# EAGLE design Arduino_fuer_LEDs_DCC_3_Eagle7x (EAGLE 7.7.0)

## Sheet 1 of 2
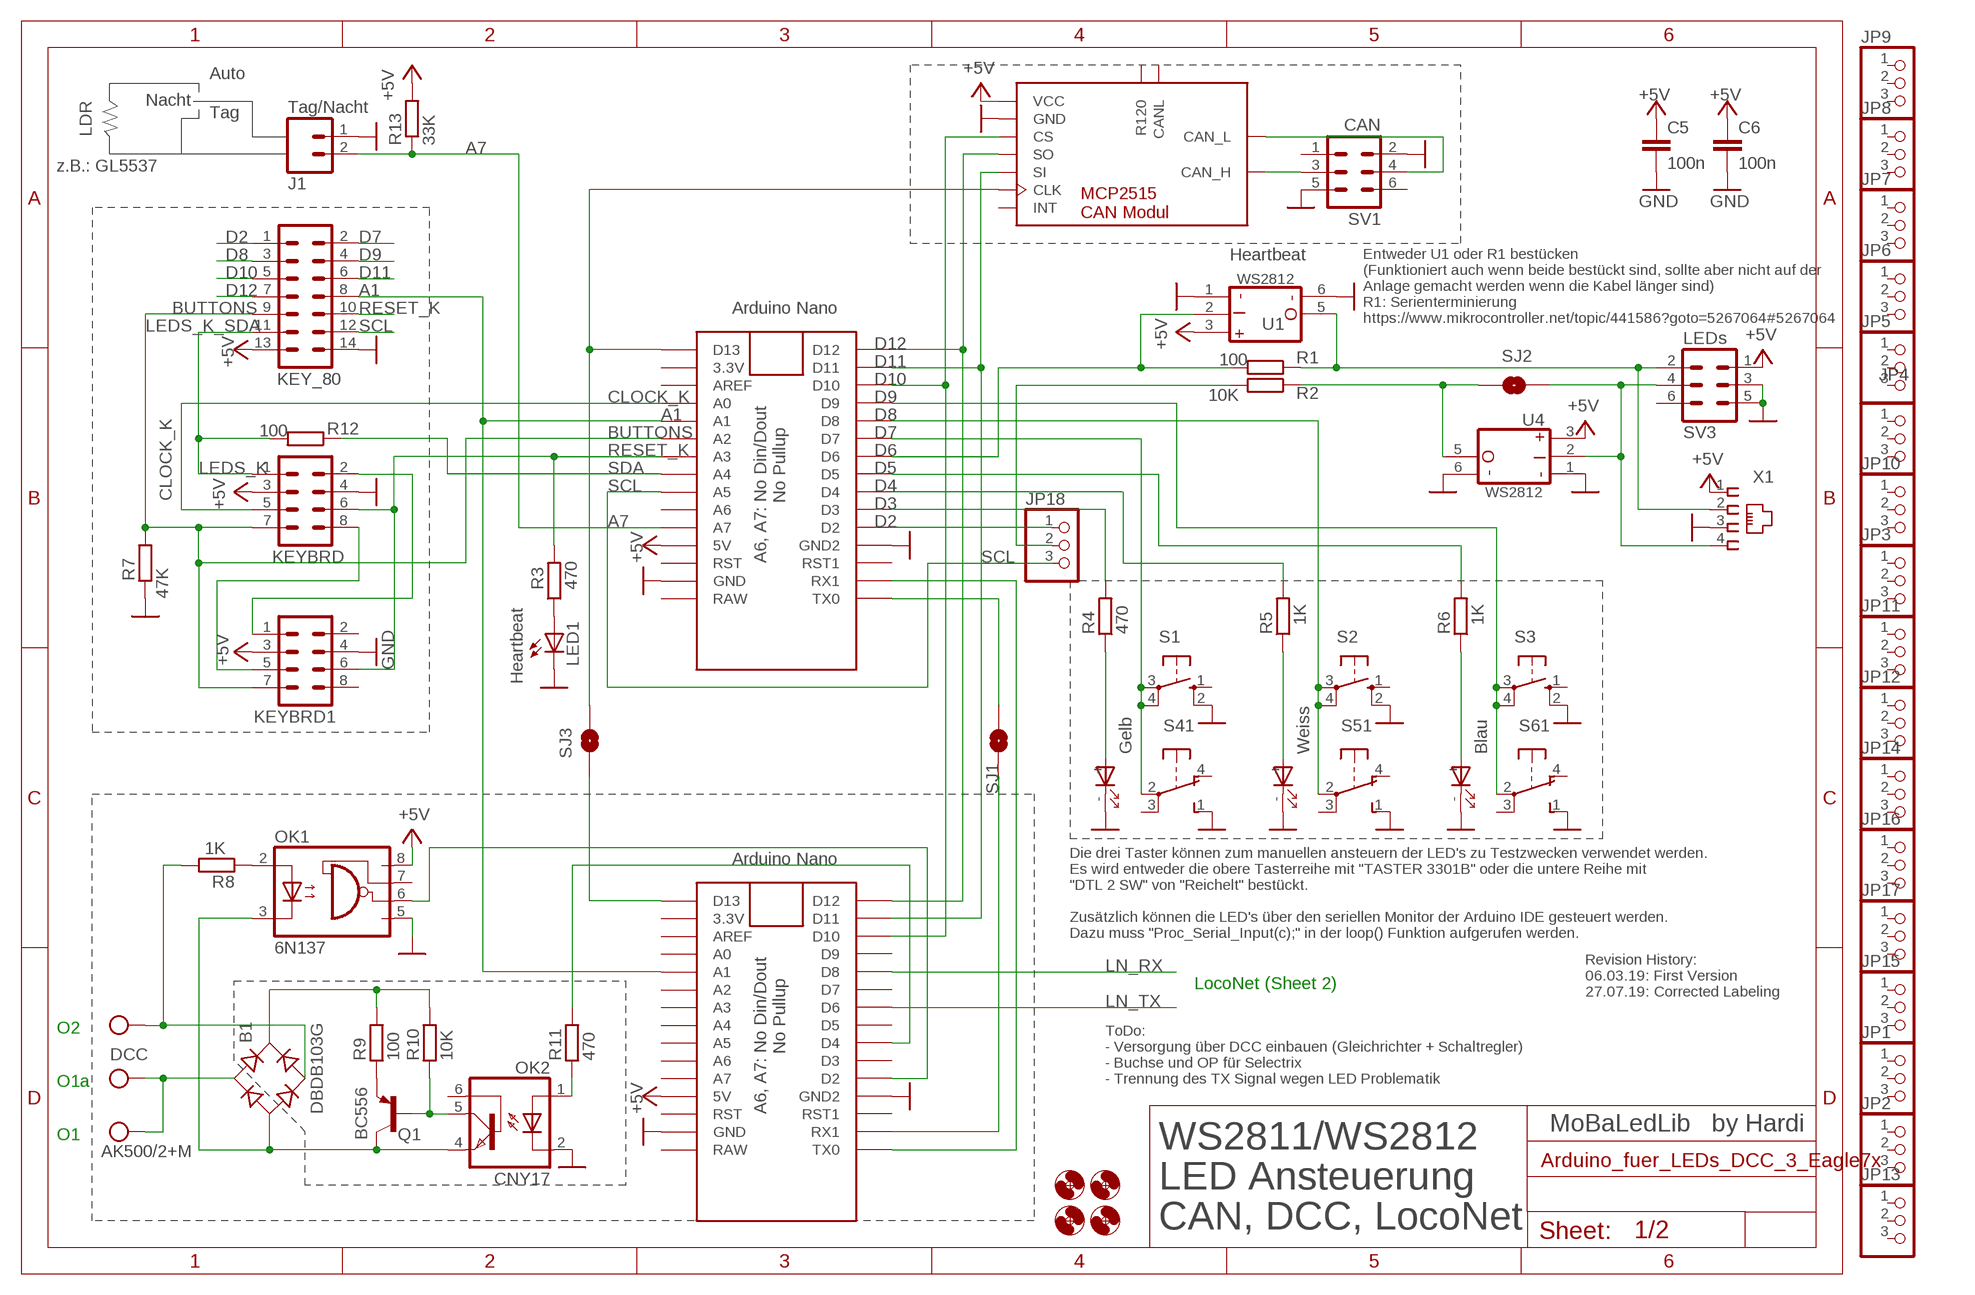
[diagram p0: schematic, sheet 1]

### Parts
B1  DBDB103G  DBDB10G  [DB]
C5  100n  C-EU025-025X050  [C025-025X050]
C6  100n  C-EU025-025X050  [C025-025X050]
CAN2  MCP2515_CAN_MODUL  [MCP2515_CAN_MODUL]
H1  MOUNT-HOLE3.0  [3,0]
H2  MOUNT-HOLE3.0  [3,0]
H3  MOUNT-HOLE3.0  [3,0]
H4  MOUNT-HOLE3.0  [3,0]
J1  Tag/Nacht  M02PTH  [1X02]
JP1  PINHD-1X3CB  [1X03-CLEANBIG]
JP2  PINHD-1X3CB  [1X03-CLEANBIG]
JP3  PINHD-1X3CB  [1X03-CLEANBIG]
JP4  PINHD-1X3CB  [1X03-CLEANBIG]
JP5  PINHD-1X3CB  [1X03-CLEANBIG]
JP6  PINHD-1X3CB  [1X03-CLEANBIG]
JP7  PINHD-1X3CB  [1X03-CLEANBIG]
JP8  PINHD-1X3CB  [1X03-CLEANBIG]
JP9  PINHD-1X3CB  [1X03-CLEANBIG]
JP10  PINHD-1X3CB  [1X03-CLEANBIG]
JP11  PINHD-1X3CB  [1X03-CLEANBIG]
JP12  PINHD-1X3CB  [1X03-CLEANBIG]
JP13  PINHD-1X3CB  [1X03-CLEANBIG]
JP14  PINHD-1X3CB  [1X03-CLEANBIG]
JP15  PINHD-1X3CB  [1X03-CLEANBIG]
JP16  PINHD-1X3CB  [1X03-CLEANBIG]
JP17  PINHD-1X3CB  [1X03-CLEANBIG]
JP18  PINHD-1X3CB  [1X03-CLEANBIG]
KEY_80  ML14  [ML14]
KEYBRD  CON-HARTING-ML_ML08  [CON-HARTING-ML_ML08]
KEYBRD1  CON-HARTING-ML_ML08  [CON-HARTING-ML_ML08]
LED1  Heartbeat  LED3MM  [LED3MM]
OK1  6N137  [DIL08]
OK2  CNY17  [DIL06]
Q1  BC556  [TO92-EBC]
R1  100  R0204/7  [0204/7]
R2  10K  R0204/7  [0204/7]
R3  470  R0204/7  [0204/7]
R4  470  R0204/7  [0204/7]
R5  1K  R0204/7  [0204/7]
R6  1K  R0204/7  [0204/7]
R7  47K  R0204/7  [0204/7]
R8  1K  R0204/7  [0204/7]
R9  100  R0204/7  [0204/7]
R10  10K  R0204/7  [0204/7]
R11  470  R0204/7  [0204/7]
R12  100  R0204/7  [0204/7]
R13  33K  R0204/7  [0204/7]
S1  10-XX  [B3F-10XX]
S2  10-XX  [B3F-10XX]
S3  10-XX  [B3F-10XX]
S4  Gelb  SRKL  [SRKL]
S5  Weiss  SRKL  [SRKL]
S6  Blau  SRKL  [SRKL]
SJ1  SOLDERJUMPERNO  [SJ_2S-NO]
SJ2  SOLDERJUMPERNO  [SJ_2S-NO]
SJ3  SOLDERJUMPERNO  [SJ_2S-NO]
SV1  CAN  ML6  [ML6]
SV3  LEDs  ML6  [ML6]
U1  WS2812_MODUL  [WS2812_LED_MODUL]
U2  LED NANO  NANO  [NANO]
U3  DCC NANO  NANO  [NANO]
U4  WS2812_MODUL  [WS2812_LED_MODUL]
X1  RJ10  [RJ10]
X2  AK500/2+M  [AK500/2+M]

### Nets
+5V: C5.1 C6.1 CAN2.1(VCC) KEY_80.13 KEYBRD1.3 KEYBRD.3 OK1.8(VCC) R13.2 SV3.1 U1.3(VDD) U2.5V U3.5V U4.3(VDD) X1.1 ; also sheet 2
A1: KEY_80.8 U2.A1 U3.A1
A7: J1.2 R13.1 U2.A7
BUTTONS: KEY_80.9 KEYBRD1.7 KEYBRD.7 R7.2 U2.A2
CAN_H: CAN2.9(CAN_H) SV1.3
CAN_L: CAN2.8(CAN_L) SV1.4
CLOCK_K: KEYBRD.5 U2.A0
D2: JP18.1 KEY_80.1 U2.D2
D3: R4.2 U2.D3
D4: R5.2 U2.D4
D5: R6.2 U2.D5
D6: R1.2 U1.2(DIN) U2.D6
D7: KEY_80.2 S1.3(P) S1.4(P1) S4.2(1:P) U2.D7
D8: KEY_80.3 S2.3(P) S2.4(P1) S5.2(1:P) U2.D8
D9: KEY_80.4 S3.3(P) S3.4(P1) S6.2(1:P) U2.D9
D10: CAN2.3(CS) KEY_80.5 U2.D10 U3.D10
D11: CAN2.5(SI) KEY_80.6 U2.D11 U3.D11
D12: CAN2.4(SO) KEY_80.7 U2.D12 U3.D12
GND: C5.2 C6.2 CAN2.2(GND) J1.1 KEY_80.14 KEYBRD1.4 KEYBRD.4 LED1.K(C) OK1.5(GND) OK2.2(C) R7.1 S1.2(S1) S2.2(S1) S3.2(S1) S4.1(1:S) S4.-(D1:C) S5.1(1:S) S5.-(D1:C) S6.1(1:S) S6.-(D1:C) SV1.2 SV1.5 SV3.3 SV3.5 U1.1(GND) U1.6(GND1) U2.GND U2.GND1(GND2) U3.GND U3.GND1(GND2) U4.1(GND) U4.6(GND1) X1.3 ; also sheet 2
LEDS_K_SDA: KEY_80.11 KEYBRD.1 R12.2
LN_RX: U3.D8 ; also sheet 2
LN_TX: U3.D6 ; also sheet 2
N$1: SJ1.2 U2.TX0
N$2: R1.1 SV3.2 U1.5(DO) X1.2
N$3: U2.RX1 U3.TX0
N$4: R4.1 S4.+(D1:A)
N$5: CAN2.6(CLK) SJ3.2 U2.D13
N$6: R5.1 S5.+(D1:A)
N$7: R6.1 S6.+(D1:A)
N$8: OK1.6(VO) U3.D2
N$9: Q1.E R9.1
N$10: OK2.5(COL) Q1.B R10.1
N$11: SJ2.1 SV3.4 U4.2(DIN) X1.4
N$12: B1.AC2 R8.2 X2.2
N$13: B1.AC1 X2.1 X2.M
N$14: B1.+ R9.2 R10.2
N$15: OK2.1(A) R11.1
N$16: R11.2 U3.D4
N$17: B1.- OK1.3(C) OK2.4(EMI) Q1.C
N$18: SJ1.1 U3.RX1
N$19: LED1.A R3.1
N$20: SJ3.1 U3.D13
N$21: OK1.2(A) R8.1
N$22: R2.1 SJ2.2 U4.5(DO)
N$24: KEYBRD1.1 KEYBRD.2
N$25: KEYBRD1.5 KEYBRD.8
N$26: JP18.2 R2.2
RESET_K: KEY_80.10 KEYBRD1.6 KEYBRD.6 R3.2 U2.A3
SCL: JP18.3 KEY_80.12 U2.A5
SDA: R12.1 U2.A4
Unconnected: CAN2.7(INT) CAN2.10(R120) CAN2.11(CANL) JP1.1 JP1.2 JP1.3 JP2.1 JP2.2 JP2.3 JP3.1 JP3.2 JP3.3 JP4.1 JP4.2 JP4.3 JP5.1 JP5.2 JP5.3 JP6.1 JP6.2 JP6.3 JP7.1 JP7.2 JP7.3 JP8.1 JP8.2 JP8.3 JP9.1 JP9.2 JP9.3 JP10.1 JP10.2 JP10.3 JP11.1 JP11.2 JP11.3 JP12.1 JP12.2 JP12.3 JP13.1 JP13.2 JP13.3 JP14.1 JP14.2 JP14.3 JP15.1 JP15.2 JP15.3 JP16.1 JP16.2 JP16.3 JP17.1 JP17.2 JP17.3 KEYBRD1.2 KEYBRD1.8 OK1.7(VE) OK2.6(BAS) S1.1(S) S2.1(S) S3.1(S) S4.3(1:P) S4.4(1:O) S5.3(1:P) S5.4(1:O) S6.3(1:P) S6.4(1:O) SV1.1 SV1.6 SV3.6 U2.3.3V U2.A6 U2.AREF U2.RAW U2.RST U2.RST1 U3.3.3V U3.A0 U3.A2 U3.A3 U3.A4 U3.A5 U3.A6 U3.A7 U3.AREF U3.D3 U3.D5 U3.D7 U3.D9 U3.RAW U3.RST U3.RST1

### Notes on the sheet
- Auto
- Nacht
- Tag
- LDR
- z.B.: GL5537
- Heartbeat
- Entweder U1 oder R1 bestücken 
  (Funktioniert auch wenn beide bestückt sind, sollte aber nicht auf der 
  Anlage gemacht werden wenn die Kabel länger sind)
  R1: Serienterminierung
  https://www.mikrocontroller.net/topic/441586?goto=5267064#5267064
- LEDS_K
- A6, A7: No Din/Dout 
              No Pullup
- Die drei Taster können zum manuellen ansteuern der LED's zu Testzwecken verwendet werden. 
  Es wird entweder die obere Tasterreihe mit "TASTER 3301B" oder die untere Reihe mit 
  "DTL 2 SW" von "Reichelt" bestückt.
  
  Zusätzlich können die LED's über den seriellen Monitor der Arduino IDE gesteuert werden. 
  Dazu muss "Proc_Serial_Input(c);" in der loop() Funktion aufgerufen werden.
- Revision History:
  06.03.19: First Version
  27.07.19: Corrected Labeling
- LocoNet (Sheet 2)
- ToDo:
  - Versorgung über DCC einbauen (Gleichrichter + Schaltregler)
  - Buchse und OP für Selectrix
  - Trennung des TX Signal wegen LED Problematik
- O2
- DCC
- O1a
- A6, A7: No Din/Dout 
              No Pullup
- MoBaLedLib   by Hardi
- O1
- WS2811/WS2812
  LED Ansteuerung
  CAN, DCC, LocoNet

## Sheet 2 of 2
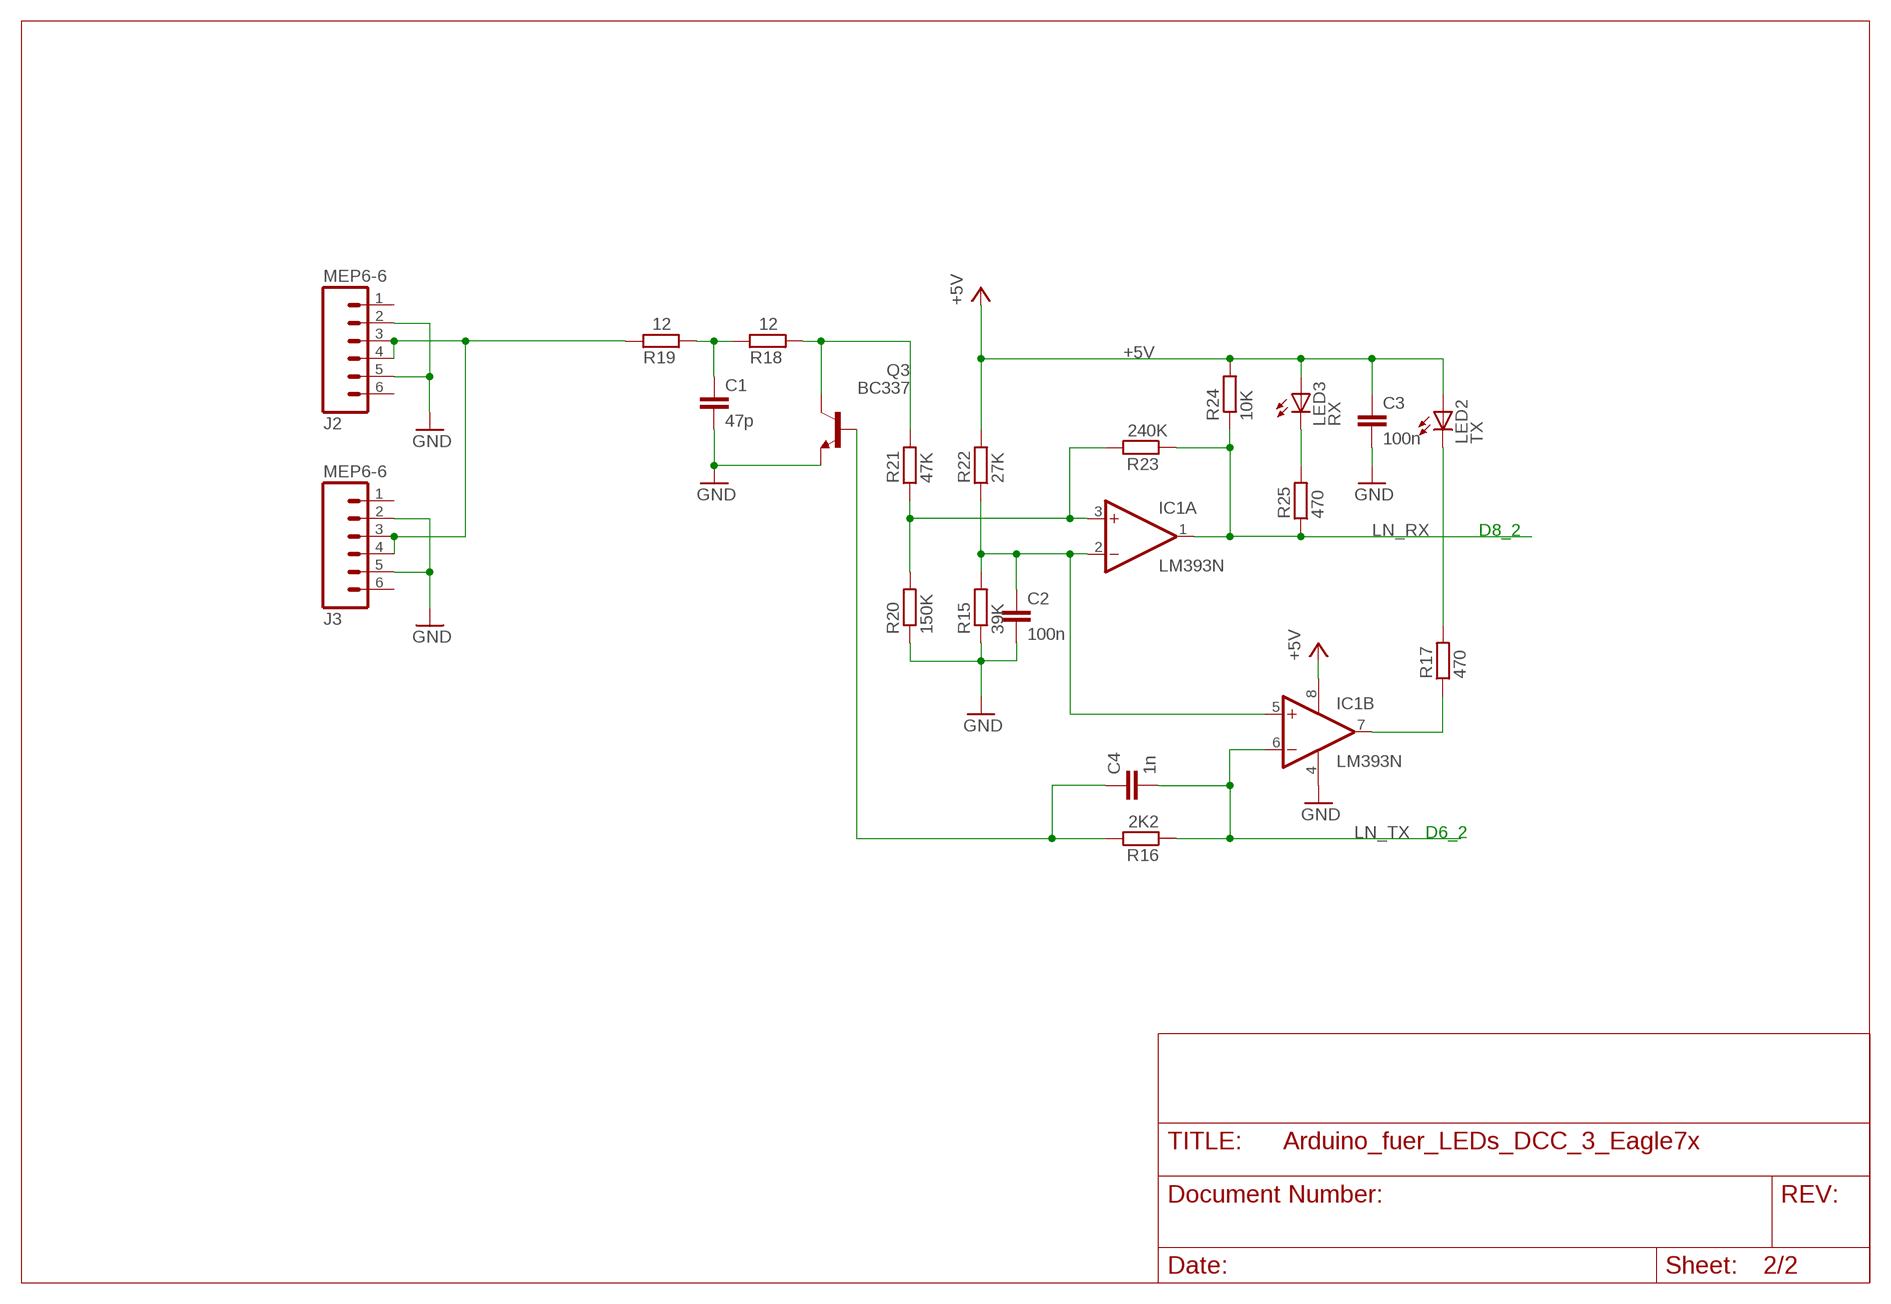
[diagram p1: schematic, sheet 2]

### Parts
C1  47p  C-EU025-025X050  [C025-025X050]
C2  100n  C-EU025-025X050  [C025-025X050]
C3  100n  C-EU025-025X050  [C025-025X050]
C4  1n  C-EU025-025X050  [C025-025X050]
IC1  LM393N  [DIL08]
J2  MEP6-6  RJ11-6PTH  [RJ11-6]
J3  MEP6-6  RJ11-6PTH  [RJ11-6]
LED2  TX  PFEIL3_LED3MM  [PFEIL3_LED3MM]
LED3  RX  PFEIL3_LED3MM  [PFEIL3_LED3MM]
Q3  BC337  [TO92]
R15  39K  R-EU_0207/2V  [0207/2V]
R16  2K2  R-EU_0207/2V  [0207/2V]
R17  470  R-EU_0207/2V  [0207/2V]
R18  12  R-EU_0207/2V  [0207/2V]
R19  12  R-EU_0207/2V  [0207/2V]
R20  150K  R-EU_0207/2V  [0207/2V]
R21  47K  R-EU_0207/2V  [0207/2V]
R22  27K  R-EU_0207/2V  [0207/2V]
R23  240K  R-EU_0207/2V  [0207/2V]
R24  10K  R-EU_0207/2V  [0207/2V]
R25  470  R-EU_0207/2V  [0207/2V]

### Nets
+5V: C3.1 IC1.8(P:V+) LED2.A LED3.A R22.2 R24.2 ; also sheet 1
GND: C1.2 C2.2 C3.2 IC1.4(P:V-) J2.2 J2.5 J3.2 J3.5 Q3.1(E) R15.1 R20.1 ; also sheet 1
LN_RX: IC1.1(A:OUT) R23.1 R24.1 R25.1 ; also sheet 1
LN_TX: C4.2 IC1.6(B:-IN) R16.1 ; also sheet 1
LOCONET: J2.3 J2.4 J3.3 J3.4 R19.1
N$31: C2.1 IC1.2(A:-IN) IC1.5(B:+IN) R15.2 R22.1
N$32: C4.1 Q3.2(B) R16.2
N$33: Q3.3(C) R18.2 R21.2
N$34: IC1.3(A:+IN) R20.2 R21.1 R23.2
N$35: IC1.7(B:OUT) R17.1
N$36: LED3.K(C) R25.2
N$37: LED2.K(C) R17.2
N$38: C1.1 R18.1 R19.2
Unconnected: J2.1 J2.6 J3.1 J3.6

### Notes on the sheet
- D8_2
- D6_2

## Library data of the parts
B1 = Arduino_fuer_LEDs_DCC_2:DB?*G: Single Phase 1.0 AMP Glass Passivated Bridge Rectifier Taiwan Semiconductor Co.,Ltd. - TSC Source: http://www.taiwansemi.com/TSCbig5/ezcatfiles/cust/img/img/db101g.pdf http://www.ts.com.tw/db/pictures/modules/PDT/PDT060207001/DBLS201G.pdf
C1-C6 = rcl:C-EU: CAPACITOR, European symbol
CAN2 = Arduino_fuer_LEDs_DCC_2_All:MCP2515_CAN_MODUL: MCP2515 CAN Modul
H1-H4 = holes:MOUNT-HOLE: MOUNTING HOLE with drill center marker
IC1 = linear:LM393: COMPARATOR
J1 = SparkFun-Connectors:M02: Standard 2-pin 0.1" header. Use with
J2 J3 = SparkFun-Connectors:RJ11-6: RJ11 Jack Simple 6 pin RJ11 jack. Commonly found on CAT3 devices and Microchip programmers. SKU: PRT-00132
JP1-JP18 = adafruit:PINHD-1X3: PIN HEADER
KEY_80 = Arduino_fuer_LEDs_DCC_2:ML14: HARTING; OC_FARNELL: unknown; OC_NEWARK: unknown
KEYBRD KEYBRD1 = PushButtonAction_4017_2:CON-HARTING-ML_ML08: Modified by Hardi; OC_FARNELL: unknown; OC_NEWARK: unknown
LED1 = Arduino_fuer_LEDs_DCC_2:LED: LED
LED2 LED3 = _relaisblock2Gl-Frontplatte:PFEIL3_LED: LED
OK1 = Arduino_fuer_LEDs_DCC_2:6N137: MOTOROLA OPTO COUPLER; MPN: 6N137; OC_FARNELL: 1328376; OC_NEWARK: 52M1895
OK2 = Arduino_fuer_LEDs_DCC_2:CNY17: SIEMENS OPTO COUPLER; MPN: CNY17-1; OC_FARNELL: 1045399; OC_NEWARK: 05M4044
Q1 = transistor-pnp:BC556*: PNP Transistror
Q3 = transistor-npn:BC337*: NPN Transistor
R1-R13 = Arduino_fuer_LEDs_DCC_2:R: RESISTOR, European symbol; SPICEMODEL: NONE; SPICEPREFIX: R
R15-R25 = rcl:R-EU_: RESISTOR, European symbol
S1-S3 = switch-omron:10-XX: OMRON SWITCH; MPN: B3F-1000; OC_FARNELL: 176432; OC_NEWARK: 36M3542
S4-S6 = switch-misc:SRKL: SWITCH
SJ1-SJ3 = SparkFun-Retired:SOLDERJUMPER: Solder Jumper
SV1 SV3 = Arduino_fuer_LEDs_DCC_2:ML6: HARTING; OC_FARNELL: unknown; OC_NEWARK: unknown
U1 U4 = Arduino_fuer_LEDs_DCC_2_All:WS2812_MODUL: WS2812 Modul mit Winkelsteckern (by Hardi)
U2 U3 = Arduino_fuer_LEDs_DCC_2:NANO: Arduino Nano
X1 = RJ10:RJ10: RJ10 Connector "C:\Dat\Märklin\Schaltpläne\Allgemein\RJ10_Stecker_Layout.docx" ...; OC_FARNELL: unknown; OC_NEWARK: unknown
X2 = Arduino_fuer_LEDs_DCC_2:AK500/2+M

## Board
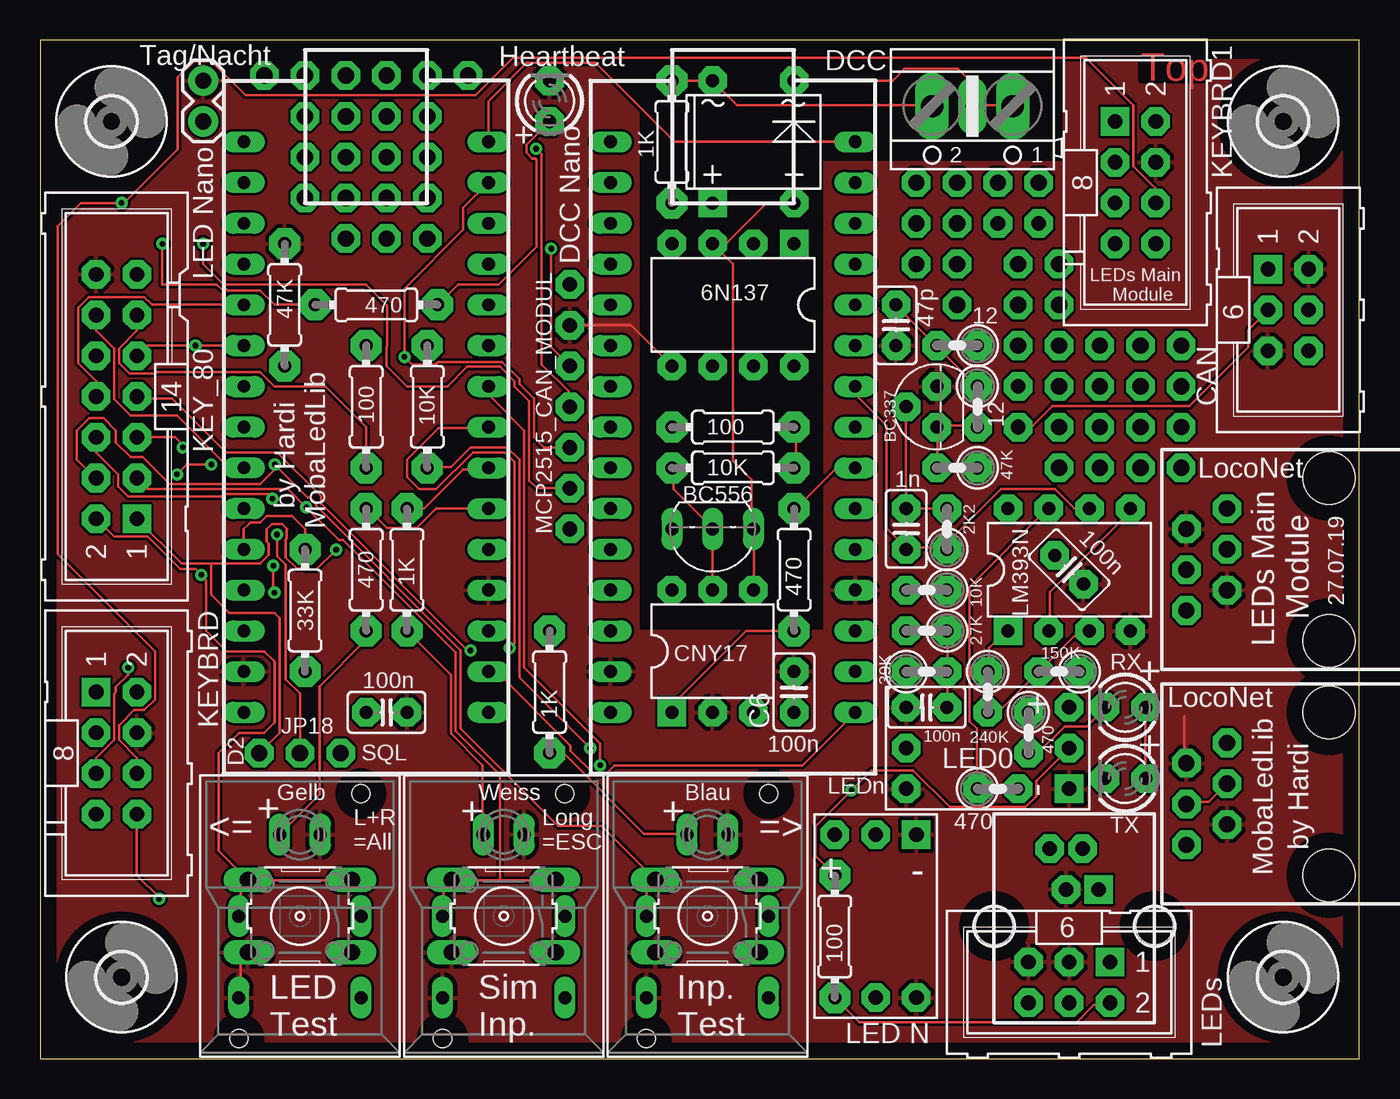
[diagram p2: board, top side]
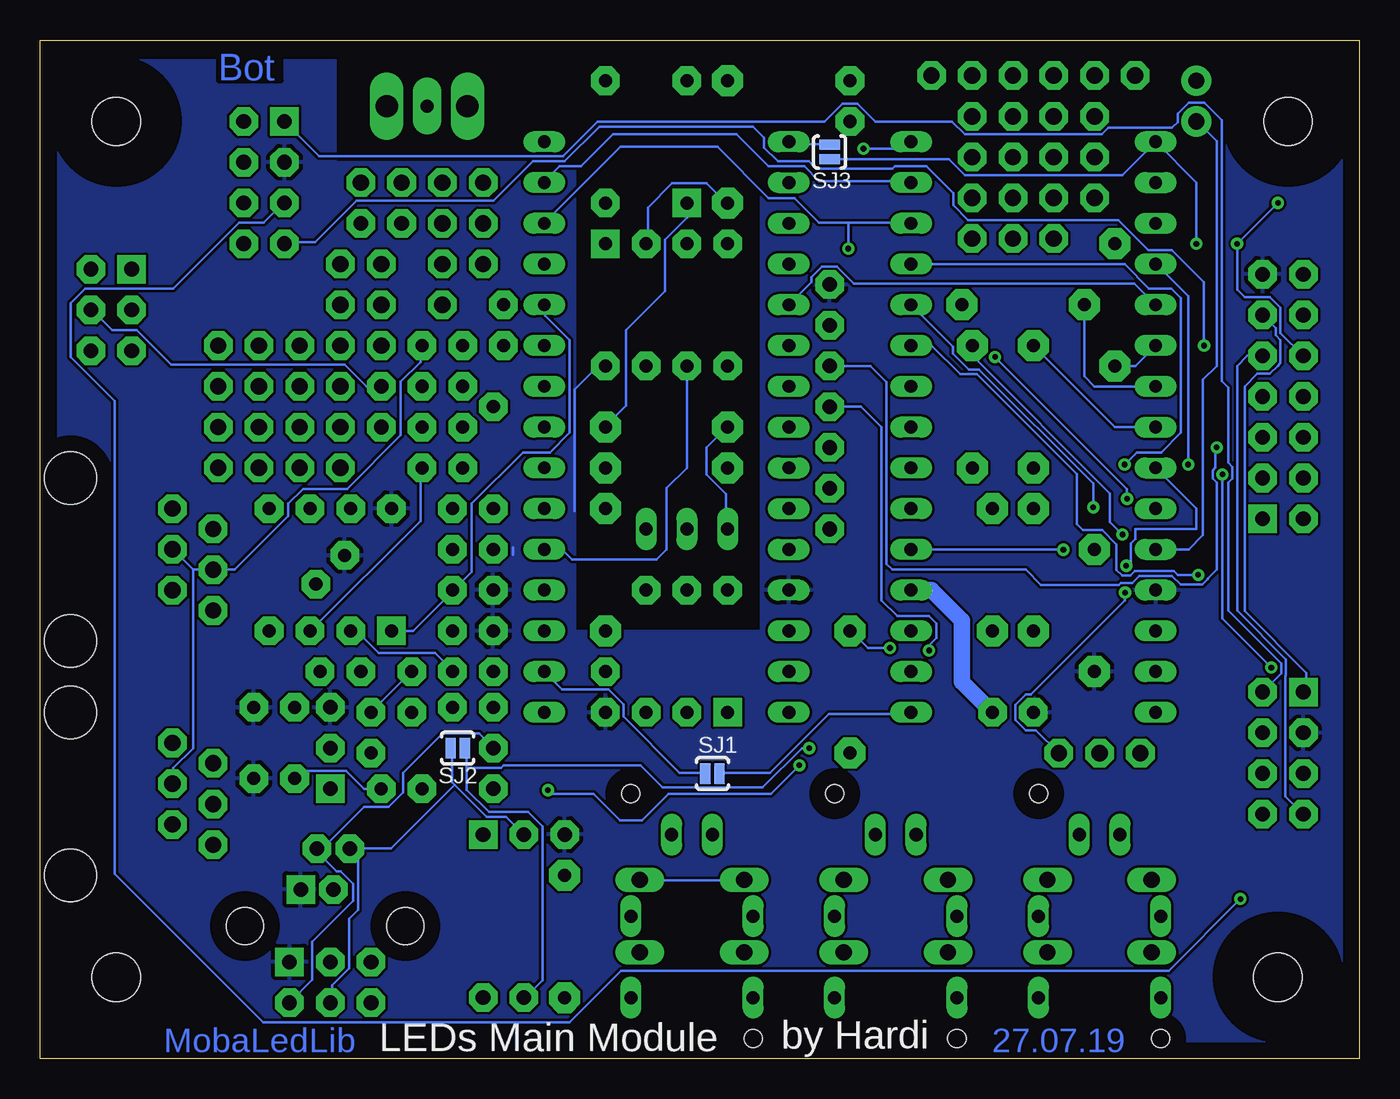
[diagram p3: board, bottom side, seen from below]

Size 82.22 x 63.49 mm. Coordinates in mm from the lower left corner, seen from the top.
Outline: 0,0 82.22,0 82.22,63.49 0,63.49 0,0
Copper layers (1*16): Top 0.035mm / dielectric 1.5mm / Bottom 0.035mm
Design rules "default": minimum track width 6mil, minimum drill 0.35mm, track to track 6mil, track to pad 6mil, pad to pad 6mil, via to via 6mil, smd to smd 6mil, copper to edge 40mil, drill to drill 6mil, minimum pad ring 10mil, minimum via ring 8mil, stop-mask expansion 4mil, vias tented up to drill 0mil, thermal gap 10mil

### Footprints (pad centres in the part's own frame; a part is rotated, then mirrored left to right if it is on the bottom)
DB = drill 0.813 pad 1.778 square: + -2.54,-3.81 | drill 0.813 pad 1.778 octagon: - 2.54,-3.81; AC1 2.54,3.81; AC2 -2.54,3.81
C025-025X050 = drill 0.813 pad 1.778 octagon: 1 -1.27,0; 2 1.27,0
MCP2515_CAN_MODUL = drill 0.914 pad 1.778 octagon: 1 0,0; 2 0,-2.54; 3 0,-5.08; 4 0,-7.62; 5 0,-10.16; 6 0,-12.7; 7 0,-15.24; 8 27.94,-6.35; 9 27.94,-8.89; 10 26.67,3.81; 11 29.21,3.81
3,0 = hole 3: 0,0
DIL08 = drill 0.813 pad 1.778 square: 1 -3.81,-3.81 | drill 0.813 pad 1.778 octagon: 2 -1.27,-3.81; 3 1.27,-3.81; 4 3.81,-3.81; 5 3.81,3.81; 6 1.27,3.81; 7 -1.27,3.81; 8 -3.81,3.81
1X02 = drill 1.016 pad 1.88: 1 0,0; 2 2.54,0
RJ11-6 = drill 1.016 pad 1.778 octagon: 1 1.905,8.89; 2 3.175,6.35; 3 4.445,8.89; 4 5.715,6.35; 5 6.985,8.89; 6 8.255,6.35 | hole 3.251: 0,0; 10.16,0
1X03-CLEANBIG = drill 1.016 pad 1.778 octagon: 1 -2.54,0; 2 0,0; 3 2.54,0
ML14 = drill 0.914 pad 1.778 square: 1 -7.62,-1.27 | drill 0.914 pad 1.778 octagon: 2 -7.62,1.27; 3 -5.08,-1.27; 4 -5.08,1.27; 5 -2.54,-1.27; 6 -2.54,1.27; 7 0,-1.27; 8 0,1.27; 9 2.54,-1.27; 10 2.54,1.27; 11 5.08,-1.27; 12 5.08,1.27; 13 7.62,-1.27; 14 7.62,1.27
CON-HARTING-ML_ML08 = drill 0.914 pad 1.778 square: 1 -5.08,-1.27 | drill 0.914 pad 1.778 octagon: 2 -5.08,1.27; 3 -2.54,-1.27; 4 -2.54,1.27; 5 0,-1.27; 6 0,1.27; 7 2.54,-1.27; 8 2.54,1.27
LED3MM = drill 0.813 pad 1.778 octagon: A -1.27,0; K 1.27,0
PFEIL3_LED3MM = drill 0.813 pad 1.778 octagon: A -1.27,0; K 1.27,0
DIL06 = drill 0.813 pad 1.778 square: 1 -2.54,-3.81 | drill 0.813 pad 1.778 octagon: 2 0,-3.81; 3 2.54,-3.81; 4 2.54,3.81; 5 0,3.81; 6 -2.54,3.81
TO92-EBC = drill 0.813 long: B 0,-1.27; C -2.54,-1.27; E 2.54,-1.27
TO92 = drill 0.813 pad 1.778 octagon: 1 1.27,0; 2 0,1.905; 3 -1.27,0
0204/7 = drill 0.813 pad 1.93 octagon: 1 -3.81,0; 2 3.81,0
0207/2V = drill 0.813 pad 1.778 octagon: 1 -1.27,0; 2 1.27,0
B3F-10XX = drill 1.016 long: 1 -3.251,2.261; 2 3.251,2.261; 3 -3.251,-2.261; 4 3.251,-2.261
SRKL = drill 0.813 long: 1 -3.81,-5.08; 2 -3.81,0; 3 3.81,0; 4 3.81,-5.08; + -1.27,5.08; - 1.27,5.08 | hole 1.118: 3.81,7.62; -3.81,-7.62
SJ_2S-NO = smd 0.635 x 1.27: 1 -0.45,0; 2 0.45,0
ML6 = drill 0.914 pad 1.778 square: 1 -2.54,-1.27 | drill 0.914 pad 1.778 octagon: 2 -2.54,1.27; 3 0,-1.27; 4 0,1.27; 5 2.54,-1.27; 6 2.54,1.27
WS2812_LED_MODUL = drill 0.914 pad 1.778 square: 1 -5.08,-5.08 | drill 0.914 pad 1.778 octagon: 2 -2.54,-5.08; 3 0,-5.08; 5 -2.54,5.08; 6 -5.08,5.08
NANO = drill 0.8 long: 3.3V -10.16,24.13; 5V -10.16,-1.27; A0 -10.16,19.05; A1 -10.16,16.51; A2 -10.16,13.97; A3 -10.16,11.43; A4 -10.16,8.89; A5 -10.16,6.35; A6 -10.16,3.81; A7 -10.16,1.27; AREF -10.16,21.59; D2 5.08,1.27; D3 5.08,3.81; D4 5.08,6.35; D5 5.08,8.89; D6 5.08,11.43; D7 5.08,13.97; D8 5.08,16.51; D9 5.08,19.05; D10 5.08,21.59; D11 5.08,24.13; D12 5.08,26.67; D13 -10.16,26.67; GND -10.16,-6.35; GND1 5.08,-1.27; RAW -10.16,-8.89; RST -10.16,-3.81; RST1 5.08,-3.81; RX1 5.08,-6.35; TX0 5.08,-8.89
RJ10 = drill 0.9 pad 1.778 square: 1 -1.524,-2.3 | drill 0.9 pad 1.778 octagon: 2 -0.508,-4.84; 3 0.508,-2.3; 4 1.524,-4.84 | hole 2.3: 5,0; -5,0
AK500/2+M = drill 1.397 long: 1 -2.515,0; 2 2.515,0 | drill 0.813 pad 1.778 long: M 0,0

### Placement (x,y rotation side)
B1  44.45,57.15 0 top
C1  53.34,45.72 270 top
C2  55.24,21.91 180 top
C3  64.14,30.48 315 top
C4  53.98,33.02 270 top
C5  21.59,21.59 0 top
C6  46.99,22.86 90 top
CAN2  33.02,48.26 0 top
H1  5.08,5.08 0 top
H2  4.45,58.42 0 top
H3  77.47,58.42 0 top
H4  77.47,5.08 0 top
IC1  64.14,30.48 0 top
J1  10.16,60.96 270 top
J2  80.33,11.43 90 top
J3  80.33,26.04 90 top
JP1  68.58,44.45 0 top
JP2  68.58,41.91 0 top
JP3  68.58,39.37 0 top
JP4  68.58,36.83 0 top
JP5  63.5,39.37 90 top
JP6  63.5,46.99 90 top
JP7  57.15,49.53 90 top
JP8  60.96,46.99 90 top
JP9  54.61,52.07 90 top
JP10  59.69,54.61 0 top
JP11  24.13,56.2 90 top
JP12  21.59,56.2 90 top
JP13  19.05,56.2 90 top
JP14  21.59,51.12 0 top
JP15  16.51,56.2 90 top
JP16  16.51,61.28 180 top
JP17  24.13,61.28 0 top
JP18  16.19,19.05 0 top
KEY_80  4.76,41.27 90 top
KEYBRD  4.76,17.78 270 top
KEYBRD1  68.26,53.34 270 top
LED1  31.75,59.69 90 top
LED2  67.63,17.46 180 top
LED3  67.63,21.91 180 top
OK1  43.18,46.99 180 top
OK2  41.91,25.4 0 top
Q1  41.91,31.75 180 top
Q3  55.88,40.64 90 top
R1  49.53,7.62 90 top
R2  24.13,40.64 90 top
R3  20.95,46.99 180 top
R4  20.32,30.48 90 top
R5  22.86,30.48 90 top
R6  31.75,22.86 90 top
R7  15.24,46.99 270 top
R8  39.37,57.15 90 top
R9  43.18,39.37 0 top
R10  43.18,36.83 0 top
R11  46.99,30.48 90 top
R12  20.32,40.64 270 top
R13  16.51,27.94 270 top
R15  55.24,24.13 0 top
R16  56.52,33.02 90 top
R17  59.69,16.83 0 top
R18  58.42,40.64 270 top
R19  57.15,44.45 180 top
R20  63.5,24.13 180 top
R21  57.15,36.83 180 top
R22  55.24,26.67 180 top
R23  59.05,22.86 270 top
R24  55.24,29.21 180 top
R25  61.59,20.32 270 top
S1  16.19,8.89 180 top
S2  28.89,8.89 180 top
S3  41.59,8.89 180 top
S4  16.19,8.89 0 top
S5  28.89,8.89 0 top
S6  41.59,8.89 0 top
SJ1  40.32,17.78 0 bottom
SJ2  56.2,19.37 0 bottom
SJ3  33.02,56.52 270 bottom
SV1  77.79,46.67 270 top
SV3  64.14,4.76 180 top
U1  59.05,21.91 90 top
U2  22.86,30.48 0 top
U3  45.72,30.48 0 top
U4  49.53,8.89 180 top
X1  64.45,8.26 180 top
X2  58.1,59.37 180 top

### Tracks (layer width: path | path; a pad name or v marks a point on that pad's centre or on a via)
+5V
  Top 0.152: LED2.A 68.89,17.53 68.89,21.79 LED3.A
  Bottom 0.152: 64.16,21.79 U1.3 | OK1.8 47.45,43.18 48.92,41.71 48.92,34.14 | 52.73,31.39 52.73,31.85
  pour Bottom: 1.27,0 81.28,0 81.28,62.23 63.82,62.23 63.82,55.88 48.9,55.88 48.9,26.67 37.31,26.67 37.31,62.23 0,62.23 0,1.27
A1
  Top 0.152: U2.A1 6.98,46.99 6.5,47.47 3.03,47.47 2.38,46.82 2.38,43.35 3.49,42.23 KEY_80.8
  Bottom 0.152: U2.A1 14.02,48.31 31.49,48.31 32.56,49.38 33.48,49.38 34.14,48.72 34.14,48.41 U3.A1
A7
  Top 0.152: U2.A7 12.7,33.02 13.02,33.34 13.09,33.41 13.72,33.41 14.13,33.81 15.72,33.81 16.51,33.02 R13.1
  Bottom 0.152: J1.2 10.06,58.37 8.89,57.2 8.89,43.18 9.75,42.32 9.75,32.63 10.64,31.75 U2.A7
BUTTONS  (via drill 0.35)
  Top 0.152: U2.A2 v9.68,44.45 6.67,44.45 KEY_80.9
  Bottom 0.152: KEYBRD1.7 66.9,50.9 65.08,50.9 62.48,53.49 53.95,53.49 51.51,55.93 49.53,55.93 47.36,58.1 37.78,58.1 37.1,57.42 37.1,56.78 36.24,55.93 34.29,55.93 33.83,55.47 29.11,55.47 28.96,55.63 26.98,55.63 25.3,53.95 25.3,53.19 24.38,52.27 15.03,52.27 13.16,50.41 11.68,50.41 9.68,48.42 v9.68,44.45 | R7.2 13.97,43.18 U2.A2 | KEYBRD.7 4.61,16.36 4.61,23.85 4.58,23.89 4.58,24.89 7.62,27.94 7.62,43.18 6.99,43.81 KEY_80.9
CAN_H
  Top 0.152: CAN2.9 60.96,39.47 61.87,39.47 63.09,40.69 71.63,40.69 75.29,44.35 75.29,45.41 76.5,46.63 SV1.3
CAN_L
  Bottom 0.152: CAN2.8 61.87,41.91 63.25,43.28 74.07,43.28 76.2,45.41 77.72,45.41 78.94,46.63 SV1.4
CLOCK_K  (via drill 0.35)
  Top 0.152: v10.67,37.03 9.14,37.03 v8.53,36.42 | v5.49,24.38 5.49,23.93 4.72,23.16 4.72,22.86 4.61,22.75 4.61,19.86 3.5,18.75 3.5,17.83 KEYBRD.5
  Bottom 0.152: v10.67,37.03 10.67,47.55 12.65,49.53 U2.A0 | v8.53,36.42 8.53,27.43 v5.49,24.38
D2  (via drill 0.35)
  Top 0.152: v18.45,31.73 17.2,30.48 16.51,30.48 16.43,30.56 16.02,30.56 15.32,31.26 15.32,32.37 15.37,32.42 15.37,32.99 15.4,33.02 15.08,33.34 14.45,33.34 14.13,33.02 14.13,32.22 14.24,32.12 14.24,31.38 13.72,30.87 10.64,30.87 | KEY_80.1 8.82,30.87 10.64,30.87 | 10.64,30.87 10.65,30.85 10.65,28.93 11.8,27.78 14.61,27.78 14.92,27.46 14.92,20.32 JP18.1
  Bottom 0.152: v18.45,31.73 18.47,31.75 U2.D2
D3
  Top 0.152: U2.D3 24.69,34.29 23.47,33.07 21.64,33.07 20.42,34.29 R4.2
D4
  Top 0.152: R5.2 23.93,34.29 26.36,36.73 27.89,36.73 U2.D4
D5  (via drill 0.35)
  Top 0.152: v29.26,25.6 29.57,25.91 29.57,37.19 28.96,37.8 26.98,37.8 24.69,35.51 23.62,35.51 22.86,36.27 22.86,37.34 24.84,39.32 27.89,39.32 U2.D5
  Bottom 0.152: v29.26,25.6 30.63,25.6 31.7,26.67 R6.2
D6  (via drill 0.35)
  Top 0.152: v34.9,18.29 34.9,19.66 30.18,24.38 30.18,39.17 28.04,41.3 28.04,41.91 U2.D6 | R1.2 48.31,12.65 48.31,14.48 v50.57,16.74 51.82,17.98 54.41,17.98 56.69,15.7 61.41,15.7 62.08,16.36 62.08,17.31 U1.2
  Bottom 0.152: v34.9,18.29 36.68,16.51 43.07,16.51 44.72,14.86 46.09,14.86 47.74,16.51 50.34,16.51 v50.57,16.74
D7  (via drill 0.35)
  Top 0.152: S4.2 12.5,8.99 12.5,10.82 12.8,11.12 S1.4 | S1.4 12.8,11.28 11.12,12.95 11.12,19.05 12.39,20.32 13.97,20.32 14.62,20.97 14.62,24.75 13.97,25.4 11.62,25.4 10.35,26.67 10.35,29.82 10,30.16 v10.04,30.16 9.68,30.52 8.73,30.52 6.72,32.54 4.61,32.54 KEY_80.2 | S1.4 12.95,11.12 19.36,11.12 S1.3
  Bottom 0.152: v10.04,30.16 11.32,30.16 11.55,30.4 14,30.4 14.28,30.12 14.78,30.12 15.14,30.47 15.14,32.07 16.02,32.94 17.23,32.94 17.62,33.34 17.62,36.44 23.84,42.66 24.88,42.66 26.67,44.45 U2.D7
D8  (via drill 0.35)
  Top 0.152: S5.2 25.15,8.99 25.15,10.67 25.6,11.12 S2.4 25.76,11.12 28.65,11.12 | 28.65,11.12 32,11.12 S2.3 | KEY_80.3 6.1,36.12 6.71,35.51 15.45,35.51 v16.59,34.37 18.63,32.33 18.89,32.33 25.91,25.31 25.91,20.42 28.65,17.68 28.65,11.12
  Bottom 0.152: v16.59,34.37 16.59,35.84 23.71,42.96 24.35,42.96 25.32,43.94 25.32,44.37 U2.D8
D9  (via drill 0.35)
  Top 0.152: 37.8,10.67 37.8,8.99 S6.2 | 37.8,10.67 38.25,11.12 S3.4 | KEY_80.4 3.35,36.27 2.29,37.34 2.29,39.17 3.05,39.93 3.96,39.93 4.72,39.17 4.72,38.41 5.64,37.49 6.4,37.49 8.08,35.81 13.72,35.81 14.63,36.73 v14.63,37.03 16.69,34.98 16.84,34.98 17.2,34.62 17.2,34.47 26.21,25.45 26.21,20.57 32.28,14.5 34.99,14.5 S3.4 | 37.8,10.67 S3.4
  Bottom 0.152: S3.3 44.81,11.12 38.41,11.12 S3.4 | U2.D9 14.63,49.53 13.11,48.01 11.73,48.01 11.12,47.4 11.12,39.01 12.34,37.8 13.87,37.8 v14.63,37.03
D10  (via drill 0.35)
  Top 0.152: v31.85,50.49 31.85,44.35 CAN2.3 | KEY_80.5 8.41,38.73 8.89,38.26 v8.89,38.1
  Bottom 0.152: 31.85,52.12 33.68,52.12 35.2,53.65 36.83,53.65 40.02,56.83 46.04,56.83 U3.D10 | 31.85,52.12 28.04,52.12 U2.D10 | v31.85,50.49 31.85,52.12 | v8.89,38.1 8.97,38.02 8.97,36.85 9.14,36.67 9.14,36.17 8.89,35.92 8.89,30.48 9.44,29.93 9.44,29.91 9.79,29.56 11.14,29.56 11.68,30.09 13.72,30.09 14.15,29.66 14.86,29.66 14.99,29.53 19.84,29.53 20.8,30.48 29.11,30.48 29.48,30.85 29.48,42.18 30.48,43.18 CAN2.3
D11  (via drill 0.35)
  Top 0.152: v14.48,34.9 14.17,35.2 11.58,35.2 11.43,35.05 5.49,35.05 4.88,35.66 4.88,36.42 3.5,37.8 3.5,38.71 KEY_80.6 | U2.D11 26.36,53.03 26.36,51.66 22.71,48.01 22.71,45.72 v22.71,43.74 23.19,43.26 24.62,43.26 24.8,43.43 26.98,43.43 28.8,43.43 29.87,42.37 29.87,42.06 30.79,41.15 30.79,38.73 31.42,38.1 CAN2.5
  Bottom 0.152: U2.D11 28.04,54.71 33.68,54.71 34.59,55.63 36.83,55.63 38.83,57.63 46.51,57.63 48.51,55.63 49.84,55.63 50.75,54.71 U3.D11 | v14.48,34.9 14.48,35.51 v22.71,43.74
D12  (via drill 0.35)
  Top 0.152: CAN2.4 32.92,40.69 32.92,41.6 31.24,43.28 31.24,56.39 v30.91,56.72 | KEY_80.7 6.1,41.15 8.23,41.15 11.58,37.8 14.78,37.8 17.5,35.08 17.5,34.59 26.64,25.45 v26.82,25.45 | U3.D12 39.53,57.15 34.6,62.08 30.33,62.08 27.94,59.69 U2.D12
  Bottom 0.152: v26.82,25.45 26.82,25.76 26.36,26.21 26.36,27.13 26.82,27.58 28.8,27.58 29.78,28.56 29.78,39.37 31.05,40.64 CAN2.4 | v30.91,56.72 28.37,56.72 U2.D12
GND
  Top 0.152: 64.77,24.23 R20.1 | 71.32,21.34 71.32,18.44 J2.5 | S4.1 12.5,3.81 12.5,6.25 12.8,6.55 S1.2 | 15.24,51.51 R7.1 | OK1.5 36.83,45.72 CAN2.2
  Bottom 1.016: U2.GND1 26.67,29.21 24.77,27.3 24.77,23.5 C5.2
  pour Top: 1.27,0 81.28,0 81.28,62.23 63.82,62.23 63.82,55.88 48.9,55.88 48.9,26.67 37.31,26.67 37.31,62.23 0,62.23 0,1.27
LEDS_K_SDA
  Top 0.152: KEY_80.11 6.03,45.4 4.92,44.28 4.92,43.35 5.57,42.7 7.14,42.7 7.23,42.79 13.72,42.79 14.6,41.91 17.78,41.91 20.32,39.37 R12.2
  Bottom 0.152: KEYBRD.1 3.31,23.05 3.31,24.06 7.15,27.9 7.15,41.91 6.36,42.7 5.57,42.7 5.09,43.18 5.08,43.18 5.08,43.19 4.92,43.35 4.92,44.81 5.22,45.11 5.22,45.54 KEY_80.11
LN_RX
  Top 0.152: R23.1 59.13,24.23 59.13,25.6 60.2,26.67 IC1.1
  Bottom 0.152: R25.1 61.57,21.64 59.13,24.08 R23.1 | U3.D8 50.75,46.94 50.75,46.33 49.23,44.81 49.23,39.01 50.44,37.8 52.12,37.8 55.32,34.59 55.32,30.33 56.39,29.26 R24.1 56.54,29.11 58.98,26.67 IC1.1
LN_TX
  Top 0.152: U3.D6 50.9,41.91 50.9,41.3 52.73,39.47 52.73,33.07 53.95,31.85 C4.2 54.1,31.85 56.24,31.85 | 56.24,31.85 56.39,31.85 R16.1 56.24,31.85 | IC1.6 64.47,34.29 63.25,35.51 59.89,35.51 56.24,31.85
LOCONET
  Top 0.152: J2.3 71.48,16 72.85,16 73.91,17.07 J2.4
  Bottom 0.152: 72.69,30.48 J3.3 70.1,30.48 66.75,33.83 66.75,34.59 65.84,35.51 63.09,35.51 59.74,38.86 59.74,42.22 58.52,43.43 58.52,44.35 R19.1 | 72.69,30.48 73.91,31.7 J3.4 | 72.69,30.48 72.69,19.36 73.91,18.14 73.91,17.22 J2.4
N$1
  Bottom 0.152: SJ1.2 39.78,17.83 36.73,17.83 33.07,21.49 28.04,21.49 U2.TX0
N$2
  Top 0.152: R1.1 51.05,2.29 64.62,2.29 65.68,3.35 66.6,3.35 SV3.2
  Bottom 0.152: 64.92,13.11 64.62,13.11 62.03,15.7 60.5,15.7 59.59,16.61 59.59,17.83 57.15,20.27 54.86,20.27 54.1,19.51 U1.5 | 64.92,13.11 X1.2 | SV3.2 65.25,4.92 65.25,7.29 62.71,9.84 62.71,10.9 63.48,11.67 63.74,11.67 64.92,12.85 64.92,13.11
N$3
  Top 0.152: U2.RX1 28.04,24.08 28.5,24.08 33.07,19.51 33.07,19.2 34.59,17.68 35.2,17.68 35.81,18.29 47.5,18.29 U3.TX0
N$4
  Top 0.152: R4.1 20.27,26.67 20.27,26.06 17.42,23.22 17.42,16.47 S4.+
N$5  (via drill 0.35)
  Top 0.152: CAN2.6 30.96,35.56 30.48,36.04 30.48,41 29.57,41.91 29.57,42.22 28.65,43.13 26.62,43.13 25.4,41.91 22.86,41.91 21.59,43.18 21.59,44.4 21.64,44.45 21.64,46.94 20.32,48.26 11.43,48.26 10.16,49.53 v10.16,50.8
  Bottom 0.152: SJ3.2 32.92,56.08 25.6,56.08 24.59,55.08 14.77,55.08 U2.D13 10.16,54.61 v10.16,50.8
N$6
  Top 0.152: R5.1 25.6,23.93 25.6,20.27 27.58,18.29 27.58,14.02 S5.+
N$7
  Top 0.152: R6.1 32.61,19.05 37.64,14.02 40.23,14.02 S6.+
N$8
  Bottom 0.152: U3.D2 49.69,31.75 49.05,31.11 43.81,31.11 43.18,31.75 43.18,35.56 41.91,36.83 OK1.6
N$9
  Bottom 0.152: Q1.E 39.47,33.07 39.47,35.2 40.69,36.42 40.69,38.1 39.47,39.32 R9.1
N$10
  Top 0.152: OK2.5 Q1.B 41.91,33.07 39.47,35.51 39.47,36.73 R10.1
N$11
  Bottom 0.152: 56.39,17.07 54.41,15.09 53.19,15.09 U4.2 | 56.39,17.07 56.54,17.22 56.54,19.36 SJ2.1 | SV3.4 64.01,3.5 64.01,4.57 62.95,5.63 62.95,8.73 62.39,9.29 62.39,12.55 62.86,13.02 X1.4 62.79,13.11 60.35,13.11 56.39,17.07
N$12
  Top 0.152: R8.2 B1.AC2 43.43,59.44 55.47,59.44 X2.2
N$13
  Top 0.152: 58.37,59.44 60.5,59.44 X2.1 | 58.37,59.44 58.22,59.44 58.17,59.41 | 58.17,59.41 X2.M 58.37,59.44 | B1.AC1 53.14,60.96 53.87,61.7 57.21,61.7 58.1,60.8 58.1,59.48 58.17,59.41
N$14
  Top 0.152: R10.2 47.09,36.88 47.09,39.32 R9.2
  Bottom 0.152: B1.+ 41.91,52.43 43.28,51.05 43.28,47.84 45.71,45.41 45.71,40.7 46.94,39.47 R9.2
N$15
  Top 0.152: OK2.1 39.37,22.05 43.99,26.67 R11.1
N$16
  Top 0.152: U3.D4 50.75,36.73 49.53,36.73 47.09,34.29 R11.2
N$17
  Top 0.152: OK2.4 44.5,29.26 44.5,32.92 Q1.C 44.35,33.07 44.35,36.1 43.18,37.27 43.18,49.53 OK1.3 41.91,50.9 42.82,50.9 45.26,53.34 B1.-
N$18
  Bottom 0.152: U3.RX1 49.68,23.01 46.79,23.01 45.87,22.1 45.87,21.34 42.37,17.83 40.84,17.83 SJ1.1
N$19
  Top 0.152: LED1.A 30.3,56.97 30.3,56.47 30.66,56.11 30.86,56.11 30.94,56.04 30.94,50.62 28.57,48.26 26.04,48.26 R3.1
N$20
  Bottom 0.152: SJ3.1 33.07,57 35.36,57 35.51,57.15 U3.D13
N$21
  Bottom 0.152: OK1.2 44.35,50.9 44.35,53.03 42.82,54.56 40.69,54.56 39.47,53.34 R8.1
N$22  (via drill 0.35)
  Top 0.152: v34.29,19.36 29.87,23.77 29.87,37.34 29.11,38.1 26.82,38.1 25.6,36.88 24.23,36.88 R2.1
  Bottom 0.152: 55.63,18.14 55.63,16.76 54.25,15.39 51.82,15.39 50.9,14.48 50.9,4.88 51.97,3.81 U4.5 | 55.63,18.14 55.63,19.36 SJ2.2 | v34.29,19.36 34.75,19.36 37.19,16.92 43.43,16.92 44.81,18.29 53.34,18.29 53.49,18.14 55.63,18.14
N$24
  Bottom 0.152: KEYBRD1.1 64.84,56.27 49.62,56.27 47.48,58.41 33.34,58.41 32.21,59.54 31.29,59.54 30.16,58.41 25.38,58.41 24.59,57.62 16.05,57.62 15.63,58.03 11.68,58.03 11.33,58.38 11.33,58.9 10.64,59.59 9.68,59.59 8.59,58.5 8.59,42.24 8.18,41.84 8.18,37.15 7.93,36.89 7.93,36.17 8.18,35.92 8.18,27.94 4.88,24.64 4.88,24.01 KEYBRD.2
N$25  (via drill 0.35)
  Top 0.152: KEYBRD.8 6.03,11.43 7.42,10.05 v7.42,9.96
  Bottom 0.152: v7.42,9.96 11.89,5.49 46.02,5.49 49.23,2.29 68.33,2.29 77.57,11.53 77.57,41 80.31,43.74 80.31,47.09 79.4,48.01 73.91,48.01 69.8,52.12 68.28,52.12 67.06,53.34 KEYBRD1.5
N$26  (via drill 0.35)
  Top 0.152: JP18.2 16.19,22.76 15.32,23.64 15.32,30.8 14.76,31.35 v14.76,32.67
  Bottom 0.152: R2.2 24.13,43.81 15.56,35.24 15.56,35.08 15.56,33.47 v14.76,32.67
N$31
  Top 0.152: C2.1 56.54,21.95 56.54,24.08 R15.2 56.54,24.23 56.54,26.67 R22.1 | IC1.5 67.82,34.29 67.82,33.98 62.94,29.11 62.94,26.67 IC1.2
  Bottom 0.152: IC1.2 62.48,26.67 61.11,25.3 57.61,25.3 56.54,24.23 R15.2
N$32
  Top 0.152: R16.2 C4.1 53.95,34.29 53.95,40.54 Q3.2
N$33
  Top 0.152: R21.2 55.93,36.88 55.93,39.32 Q3.3 55.93,39.47 58.37,39.47 R18.2
N$34
  Top 0.152: R23.2 59.13,21.64 59.74,21.64 R20.2 64.77,26.67 IC1.3
  Bottom 0.152: R21.1 58.52,36.73 58.52,33.53 65.38,26.67 IC1.3
N$35
  Top 0.152: R17.1 58.37,16.92 58.37,20.57 57.91,21.03 57.91,29.41 62.79,34.29 IC1.7
N$36
  Top 0.152: R25.2 62.18,19.05 63.86,20.73 65.23,20.73 66.29,21.79 LED3.K
N$37
  Bottom 0.152: R17.2 62.03,16.83 63.15,17.95 65.88,17.95 LED2.K
N$38
  Top 0.152: R18.1 58.37,41.91 55.93,44.35 R19.2 55.78,44.5 53.34,46.94 C1.1
RESET_K  (via drill 0.35)
  Top 0.152: KEYBRD1.6 69.49,53.34 69.49,54.25 68.12,55.63 68.12,59.44 65.16,62.4 29.48,62.4 27.13,60.05 12.8,60.05 10.67,62.18 9.6,62.18 8.59,61.16 8.59,56.7 5.22,53.34 v5.08,53.34 2.54,53.34 1.09,51.89 1.09,31.47 7.16,25.4 7.16,22.41 6.5,21.74 5.87,21.74 4.92,20.78 4.92,19.86 6.03,18.74 KEYBRD.6 | R3.2 14.6,46.99 13.72,47.87 11.68,47.87 11.6,47.95 11.3,47.95 11,48.26 7.62,48.26 v7.62,50.8
  Bottom 0.152: U2.A3 16.51,41.91 17.14,42.55 R3.2 | v5.08,53.34 v7.62,50.8 7.62,47.94 7.15,47.47 5.57,47.47 4.92,46.82 4.92,45.24 KEY_80.10
SCL  (via drill 0.35)
  Top 0.152: U2.A5 12.65,36.88 11.73,36.88 8.53,40.08 5.64,40.08 4.61,41.11 4.61,44.28 3.5,45.38 3.5,46.33 KEY_80.12 | v14.53,30.72 14.53,29.12 v14.61,29.05
  Bottom 0.152: JP18.3 20.16,20.47 20.78,20.47 21.44,21.13 21.44,22.05 20.78,22.71 20.47,22.71 14.61,28.57 v14.61,29.05 | U2.A5 10.16,34.29 10.16,33.02 13.97,33.02 13.97,32.38 14.24,32.12 14.24,30.85 14.36,30.72 v14.53,30.72
SDA
  Bottom 0.152: R12.1 15.24,39.37 U2.A4

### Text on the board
Top: Top
Bottom: Bot | 27.07.19 | MobaLedLib
tPlace: + | SQL | D2 | <= | => | L+R / =All | Long / =ESC | LED / Test | Sim / Inp. | Inp. / Test
bPlace: by Hardi | LEDs Main Module
tNames: DCC | DCC Nano | LED Nano | LEDs Main / Module | LocoNet | by Hardi | MobaLedLib | 27.07.19 | LEDs Main / Module | + | LocoNet | + | LED0 | LEDn | + | + | + | by Hardi | MobaLedLib | LED N

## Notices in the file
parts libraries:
SparkFun-Connectors: Licensing: Creative Commons ShareAlike 4.0 International - https://creativecommons.org/licenses/by-sa/4.0
